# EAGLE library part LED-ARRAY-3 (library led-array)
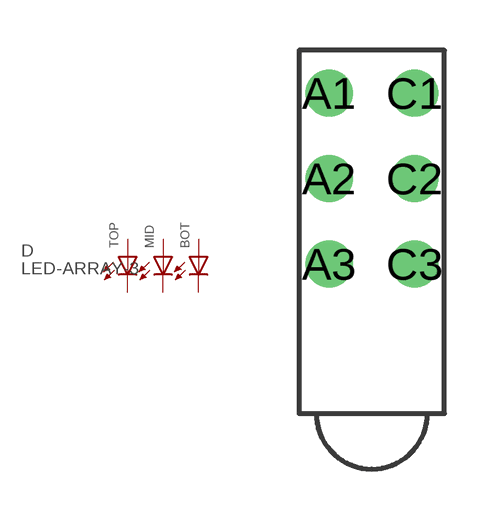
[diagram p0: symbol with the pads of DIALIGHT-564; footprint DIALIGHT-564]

Designator prefix D

## LED-ARRAY-3-564  [DIALIGHT-564]
A1  A1  pas
A2  A2  pas
A3  A3  pas
C1  C1  pas
C2  C2  pas
C3  C3  pas

## Footprint DIALIGHT-564 (pad centres in mm)
drill 0.9: A1 0,5.08; A2 0,2.54; A3 0,0; C1 2.54,5.08; C2 2.54,2.54; C3 2.54,0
